| Teraspeed Modeling Services.
| http://www.teraspeed.com
[IBIS Ver] 4.0
[File Name] ads54t01.ibs
[File Rev] 3.1
[Date]   09-17-2012
[Notes]  Quality Check of this IBIS model: Model Passes IBIS Check. Model
   parses into ICX IS. Simulates with Hyperlynx.
   1. MIN TYP MAX information is based on Temperature and Voltage
   characteristics only.
   2. Package information extracted using Tektronix IConnect Software.
[Disclaimer]
| Use: Teraspeed Consulting Group LLC ("Teraspeed") has
| licensed IBIS models to specific integrated circuit
| suppliers ("IC Vendors") for use and distribustion as
| follows: Each IC Vendor may use IBIS Models, and distribute
| them to IC Vendor's custumers to use solely for developing
| printed circute board designs. Users of this model may
| modify the IBIS model to suit its specific applications but
| rights to derivative works and such modifications shall belong
| to Teraspeed. No other distribusion of these materials is
| permitted.
| DISCLAIMER OF WARRANTY: UNLESS OTHERWISE AGREED TO IN WRITING
| TERASPEED DISCLAIMS AND USER WAIVES ALL WARRANTIES, EXPRESS
| OR IMPLIED, INCLUDING WARRANTIES OF MERCHANTABILITY AND
| FITNESS FOR A PARTICULAR PURPOSE. IN NO EVENT SHALL
| TERASPEED BE LIABLE FOR ANY DIRECT OR INDIRECT DAMAGES,
| WHETHER IN CONTRACT OR TORT, INCLUDING, WITHOUT LIMITATION,
| LOST PROFITS, BUSINESS INTERRUPTION, OR LOST INFORMATION
| ARISING OUT OF THE USE OF OR THE INABILITY TO USE THE MODEL,
| EVEN IF TERASPEED HAS BEEN ADVISED OF THE POSSIBILITY OF SUCH
| DAMAGES.
[Source]
| This model file was created by Teraspeed Consulting Group LLC
| (http://www.teraspeed.com/).
[Disclaimer]
| This product is designed as an aid for customers of Texas Instruments.
| No warranties, either expressed or implied, with respect to this third
| party software (if any) or with respect to its fitness for any
| particular purpose is claimed by Texas Instruments or the author. The
| software (if any) is provided solely on an "as is" basis. The entire
| risk as to its quality and performance is with the customer
[Copyright]
| (C) Copyright 2012 Texas Instruments Incorporated. All rights reserved.
| All other rights are reserved.
[Component] ADS54T01
[Manufacturer] TI
[Package]
| ZAY (S-PBGA-N196)
| variable   typ   min   max
R_pkg  1.000E-02   1.000E-02   1.000E-02
L_pkg  1.602E-09   1.120E-09   3.139E-09
C_pkg  7.423E-13   5.322E-13   1.384E-12
[Pin] signal_name  model_name  R_pin  L_pin C_pin
A1   DB6N   lvds_out   1.000E-02   3.139E-09   1.384E-12
A2   DB5N   lvds_out   1.000E-02   2.908E-09   1.282E-12
A3   DB4N   lvds_out   1.000E-02   2.700E-09   1.190E-12
A4   DB3N   lvds_out   1.000E-02   2.521E-09   1.111E-12
A5   DB2N   lvds_out   1.000E-02   2.378E-09   1.048E-12
A6   DB1N   lvds_out   1.000E-02   2.278E-09   1.004E-12
A7   DB0N   lvds_out   1.000E-02   2.226E-09   9.813E-13
A8   DVDD   POWER   1.000E-02   2.226E-09   9.813E-13
A9   DVDD   POWER   1.000E-02   2.278E-09   1.004E-12
A10   SDO   spi_tri   1.000E-02   2.378E-09   1.048E-12
A11   SDIO   spi_io   1.000E-02   2.521E-09   1.111E-12
A12   SCLK   in_pd   1.000E-02   2.700E-09   1.190E-12
A13   *SDEN   in_pd   1.000E-02   2.908E-09   1.282E-12
A14   VREF   term   1.000E-02   3.139E-09   1.384E-12
B1   DB6P   lvds_out   1.000E-02   2.908E-09   1.282E-12
B2   DB5P   lvds_out   1.000E-02   2.656E-09   1.171E-12
B3   DB4P   lvds_out   1.000E-02   2.427E-09   1.070E-12
B4   DB3P   lvds_out   1.000E-02   2.226E-09   9.813E-13
B5   DB2P   lvds_out   1.000E-02   2.063E-09   9.094E-13
B6   DB1P   lvds_out   1.000E-02   1.947E-09   8.581E-13
B7   DB0P   lvds_out   1.000E-02   1.886E-09   8.313E-13
B8   DVDD   POWER   1.000E-02   1.120E-09   5.620E-13
B9   DVDD   POWER   1.000E-02   1.120E-09   5.620E-13
B10   IOVDD   POWER   1.000E-02   1.120E-09   5.620E-13
B11   ENABLE   in_pu   1.000E-02   2.226E-09   9.813E-13
B12   *SRESET   in_pu   1.000E-02   2.427E-09   1.070E-12
B13   TEST_MODE   NC   1.000E-02   2.656E-09   1.171E-12
B14   VCM   term   1.000E-02   2.908E-09   1.282E-12
C1   DB7N   lvds_out   1.000E-02   2.700E-09   1.190E-12
C2   DB7P   lvds_out   1.000E-02   2.427E-09   1.070E-12
C3   DB8N   lvds_out   1.000E-02   2.173E-09   9.579E-13
C4   DB8P   lvds_out   1.000E-02   1.947E-09   8.581E-13
C5   OVRBN   lvds_out   1.000E-02   1.721E-09   7.583E-13
C6   DVDD_LVDS   POWER   1.000E-02   1.120E-09   5.620E-13
C7   DVDD_LVDS   POWER   1.000E-02   1.120E-09   5.620E-13
C8   DVDD   POWER   1.000E-02   1.120E-09   5.620E-13
C9   GND   GND   1.000E-02   1.120E-09   5.620E-13
C10   GND   GND   1.000E-02   1.120E-09   5.620E-13
C11   GND   GND   1.000E-02   1.120E-09   5.620E-13
C12   GND   GND   1.000E-02   1.120E-09   5.620E-13
C13   GND   GND   1.000E-02   1.120E-09   5.620E-13
C14   GND   GND   1.000E-02   1.120E-09   5.620E-13
D1   DB9N   lvds_out   1.000E-02   2.521E-09   1.111E-12
D2   DB9P   lvds_out   1.000E-02   2.226E-09   9.813E-13
D3   DB10N   lvds_out   1.000E-02   1.947E-09   8.581E-13
D4   DB10P   lvds_out   1.000E-02   1.690E-09   7.451E-13
D5   OVRBP   lvds_out   1.000E-02   1.433E-09   6.321E-13
D6   DVDD_LVDS   POWER   1.000E-02   1.120E-09   5.620E-13
D7   DVDD_LVDS   POWER   1.000E-02   1.120E-09   5.620E-13
D8   DVDD   POWER   1.000E-02   1.120E-09   5.620E-13
D9   GND   GND   1.000E-02   1.120E-09   5.620E-13
D10   AVDD18   POWER   1.000E-02   1.120E-09   5.620E-13
D11   AVDD18   POWER   1.000E-02   1.120E-09   5.620E-13
D12   AVDD33   POWER   1.000E-02   1.947E-09   8.581E-13
D13   GND   GND   1.000E-02   1.120E-09   5.620E-13
D14   INB_N   term   1.000E-02   2.521E-09   1.111E-12
E1   DB11N   lvds_out   1.000E-02   2.378E-09   1.048E-12
E2   DB11P   lvds_out   1.000E-02   2.063E-09   9.094E-13
E3   NC   NC   1.000E-02   1.120E-09   5.620E-13
E4   NC   NC   1.000E-02   1.120E-09   5.620E-13
E5   GND   GND   1.000E-02   1.120E-09   5.620E-13
E6   GND   GND   1.000E-02   1.120E-09   5.620E-13
E7   GND   GND   1.000E-02   1.120E-09   5.620E-13
E8   GND   GND   1.000E-02   1.120E-09   5.620E-13
E9   GND   GND   1.000E-02   1.120E-09   5.620E-13
E10   GND   GND   1.000E-02   1.120E-09   5.620E-13
E11   AVDD18   POWER   1.000E-02   1.120E-09   5.620E-13
E12   AVDD33   POWER   1.000E-02   1.120E-09   5.620E-13
E13   GND   GND   1.000E-02   1.120E-09   5.620E-13
E14   INB_P   term   1.000E-02   2.378E-09   1.048E-12
F1   SYNCOUTB_N  lvds_out   1.000E-02   2.278E-09   1.004E-12
F2   SYNCOUTB_P  lvds_out   1.000E-02   1.947E-09   8.581E-13
F3   HRESN   lvds_out   1.000E-02   1.300E-09   5.732E-13
F4   HRESP   lvds_out   1.000E-02   1.300E-09   5.732E-13
F5   GND   GND   1.000E-02   1.300E-09   5.732E-13
F6   GND   GND   1.000E-02   1.300E-09   5.732E-13
F7   GND   GND   1.000E-02   1.300E-09   5.732E-13
F8   GND   GND   1.000E-02   1.300E-09   5.732E-13
F9   GND   GND   1.000E-02   1.300E-09   5.732E-13
F10   GND   GND   1.000E-02   1.300E-09   5.732E-13
F11   AVDD18   POWER   1.000E-02   1.300E-09   5.732E-13
F12   AVDD33   POWER   1.000E-02   1.300E-09   5.732E-13
F13   GND   GND   1.000E-02   1.300E-09   5.732E-13
F14   GND   GND   1.000E-02   1.300E-09   5.732E-13
G1   DBCLKN   lvds_out   1.000E-02   2.226E-09   9.813E-13
G2   DBCLKP   lvds_out   1.000E-02   1.886E-09   8.313E-13
G3   TRDYN   lvds_out   1.000E-02   1.120E-09   5.620E-13
G4   TRDYP   lvds_out   1.000E-02   1.120E-09   5.620E-13
G5   GND   GND   1.000E-02   1.120E-09   5.620E-13
G6   GND   GND   1.000E-02   1.120E-09   5.620E-13
G7   GND   GND   1.000E-02   1.120E-09   5.620E-13
G8   GND   GND   1.000E-02   1.120E-09   5.620E-13
G9   GND   GND   1.000E-02   1.120E-09   5.620E-13
G10   GND   GND   1.000E-02   1.120E-09   5.620E-13
G11   AVDD18   POWER   1.000E-02   1.120E-09   5.620E-13
G12   AVDD33   POWER   1.000E-02   1.120E-09   5.620E-13
G13   GND   GND   1.000E-02   1.120E-09   5.620E-13
G14   AVDDC   POWER   1.000E-02   1.120E-09   5.620E-13
H1   DACLKN   lvds_out   1.000E-02   2.226E-09   9.813E-13
H2   DACLKP   lvds_out   1.000E-02   1.886E-09   8.313E-13
H3   DA0N   lvds_out   1.000E-02   1.546E-09   6.815E-13
H4   DA0P   lvds_out   1.000E-02   1.207E-09   5.322E-13
H5   GND   GND   1.000E-02   1.120E-09   5.620E-13
H6   GND   GND   1.000E-02   1.120E-09   5.620E-13
H7   GND   GND   1.000E-02   1.120E-09   5.620E-13
H8   GND   GND   1.000E-02   1.120E-09   5.620E-13
H9   GND   GND   1.000E-02   1.120E-09   5.620E-13
H10   GND   GND   1.000E-02   1.120E-09   5.620E-13
H11   AVDD18   POWER   1.000E-02   1.120E-09   5.620E-13
H12   AVDD33   POWER   1.000E-02   1.120E-09   5.620E-13
H13   GND   GND   1.000E-02   1.120E-09   5.620E-13
H14   AVDDC   POWER   1.000E-02   1.120E-09   5.620E-13
J1   DA1N   lvds_out   1.000E-02   2.278E-09   1.004E-12
J2   DA1P   lvds_out   1.000E-02   1.947E-09   8.581E-13
J3   DA2N   lvds_out   1.000E-02   1.620E-09   7.140E-13
J4   DA2P   lvds_out   1.000E-02   1.300E-09   5.732E-13
J5   GND   GND   1.000E-02   1.120E-09   5.620E-13
J6   GND   GND   1.000E-02   1.120E-09   5.620E-13
J7   GND   GND   1.000E-02   1.120E-09   5.620E-13
J8   GND   GND   1.000E-02   1.120E-09   5.620E-13
J9   GND   GND   1.000E-02   1.120E-09   5.620E-13
J10   GND   GND   1.000E-02   1.120E-09   5.620E-13
J11   AVDD18   POWER   1.000E-02   1.120E-09   5.620E-13
J12   AVDD33   POWER   1.000E-02   1.120E-09   5.620E-13
J13   GND   GND   1.000E-02   1.120E-09   5.620E-13
J14   GND   GND   1.000E-02   1.120E-09   5.620E-13
K1   DA3N   lvds_out   1.000E-02   2.378E-09   1.048E-12
K2   DA3P   lvds_out   1.000E-02   2.063E-09   9.094E-13
K3   DA4N   lvds_out   1.000E-02   1.758E-09   7.749E-13
K4   DA4P   lvds_out   1.000E-02   1.469E-09   6.474E-13
K5   GND   GND   1.000E-02   1.120E-09   5.620E-13
K6   GND   GND   1.000E-02   1.120E-09   5.620E-13
K7   GND   GND   1.000E-02   1.120E-09   5.620E-13
K8   GND   GND   1.000E-02   1.120E-09   5.620E-13
K9   GND   GND   1.000E-02   1.120E-09   5.620E-13
K10   GND   GND   1.000E-02   1.120E-09   5.620E-13
K11   AVDD18   POWER   1.000E-02   1.120E-09   5.620E-13
K12   AVDD33   POWER   1.000E-02   1.120E-09   5.620E-13
K13   GND   GND   1.000E-02   1.120E-09   5.620E-13
K14   INA_P   term   1.000E-02   2.378E-09   1.048E-12
L1   DA5N   lvds_out   1.000E-02   2.521E-09   1.111E-12
L2   DA5P   lvds_out   1.000E-02   2.226E-09   9.813E-13
L3   DA6N   lvds_out   1.000E-02   1.947E-09   8.581E-13
L4   DA6P   lvds_out   1.000E-02   1.690E-09   7.451E-13
L5   OVRAN   lvds_out   1.000E-02   1.433E-09   6.321E-13
L6   DVDD_LVDS   POWER   1.000E-02   1.120E-09   5.620E-13
L7   DVDD_LVDS   POWER   1.000E-02   1.120E-09   5.620E-13
L8   DVDD   POWER   1.000E-02   1.120E-09   5.620E-13
L9   GND   GND   1.000E-02   1.120E-09   5.620E-13
L10   AVDD18   POWER   1.000E-02   1.120E-09   5.620E-13
L11   AVDD18   POWER   1.000E-02   1.120E-09   5.620E-13
L12   AVDD33   POWER   1.000E-02   1.120E-09   5.620E-13
L13   GND   GND   1.000E-02   1.120E-09   5.620E-13
L14   INA_N   term   1.000E-02   2.521E-09   1.111E-12
M1   DA7N   lvds_out   1.000E-02   2.700E-09   1.190E-12
M2   DA7P   lvds_out   1.000E-02   2.427E-09   1.070E-12
M3   DA8N   lvds_out   1.000E-02   2.173E-09   9.579E-13
M4   DA8P   lvds_out   1.000E-02   1.947E-09   8.581E-13
M5   OVRAP   lvds_out   1.000E-02   1.721E-09   7.583E-13
M6   DVDD_LVDS   POWER   1.000E-02   1.120E-09   5.620E-13
M7   DVDD_LVDS   POWER   1.000E-02   1.120E-09   5.620E-13
M8   DVDD   POWER   1.000E-02   1.120E-09   5.620E-13
M9   GND   GND   1.000E-02   1.120E-09   5.620E-13
M10   GND   GND   1.000E-02   1.120E-09   5.620E-13
M11   GND   GND   1.000E-02   1.120E-09   5.620E-13
M12   GND   GND   1.000E-02   1.120E-09   5.620E-13
M13   GND   GND   1.000E-02   1.120E-09   5.620E-13
M14   GND   GND   1.000E-02   1.120E-09   5.620E-13
N1   DA9N   lvds_out   1.000E-02   2.908E-09   1.282E-12
N2   DA10N   lvds_out   1.000E-02   2.656E-09   1.171E-12
N3   DA11N   lvds_out   1.000E-02   2.427E-09   1.070E-12
N4   NC   NC   1.000E-02   1.120E-09   5.620E-13
N5   SYNCOUTA_N  lvds_out   1.000E-02   2.063E-09   9.094E-13
N6   HRESN   lvds_out   1.000E-02   1.120E-09   5.620E-13
N7   TRDYN   lvds_out   1.000E-02   1.120E-09   5.620E-13
N8   DVDD   POWER   1.000E-02   1.120E-09   5.620E-13
N9   SYNCN   sync_in   1.000E-02   1.947E-09   8.581E-13
N10   TRIGGERN   sync_in   1.000E-02   1.120E-09   5.620E-13
N11   AVDD18   POWER   1.000E-02   1.120E-09   5.620E-13
N12   AVDD33   POWER   1.000E-02   1.120E-09   5.620E-13
N13   GND   GND   1.000E-02   1.120E-09   5.620E-13
N14   GND   GND   1.000E-02   1.120E-09   5.620E-13
P1   DA9P   lvds_out   1.000E-02   3.139E-09   1.384E-12
P2   DA10P   lvds_out   1.000E-02   2.908E-09   1.282E-12
P3   DA11P   lvds_out   1.000E-02   2.700E-09   1.190E-12
P4   NC   NC   1.000E-02   1.120E-09   5.620E-13
P5   SYNCOUTA_P  lvds_out   1.000E-02   2.378E-09   1.048E-12
P6   HRESP   lvds_out   1.000E-02   1.120E-09   5.620E-13
P7   TRDYP   lvds_out   1.000E-02   1.120E-09   5.620E-13
P8   DVDD   POWER   1.000E-02   1.120E-09   5.620E-13
P9   SYNCP   sync_in   1.000E-02   2.278E-09   1.004E-12
P10   TRIGGERP   sync_in   1.000E-02   1.120E-09   5.620E-13
P11   AVDD18   POWER   1.000E-02   1.120E-09   5.620E-13
P12   AVDD33   POWER   1.000E-02   1.120E-09   5.620E-13
P13   CLKIN_N   clk_in   1.000E-02   2.908E-09   1.282E-12
P14   CLKIN_P   clk_in   1.000E-02   3.139E-09   1.384E-12
[Diff Pin] inv_pin vdiff tdelay_typ tdelay_min tdelay_max
B1   A1   NA   100ps   NA   NA
B2   A2   NA   100ps   NA   NA
B3   A3   NA   100ps   NA   NA
B4   A4   NA   100ps   NA   NA
B5   A5   NA   100ps   NA   NA
B6   A6   NA   100ps   NA   NA
B7   A7   NA   100ps   NA   NA
C2   C1   NA   100ps   NA   NA
C4   C3   NA   100ps   NA   NA
D5   C5   NA   100ps   NA   NA
D2   D1   NA   100ps   NA   NA
D4   D3   NA   100ps   NA   NA
E2   E1   NA   100ps   NA   NA
F2   F1   NA   100ps   NA   NA
G2   G1   NA   100ps   NA   NA
H2   H1   NA   100ps   NA   NA
H4   H3   NA   100ps   NA   NA
J2   J1   NA   100ps   NA   NA
J4   J3   NA   100ps   NA   NA
K2   K1   NA   100ps   NA   NA
K4   K3   NA   100ps   NA   NA
L2   L1   NA   100ps   NA   NA
L4   L3   NA   100ps   NA   NA
M5   L5   NA   100ps   NA   NA
M2   M1   NA   100ps   NA   NA
M4   M3   NA   100ps   NA   NA
P1   N1   NA   100ps   NA   NA
P2   N2   NA   100ps   NA   NA
P3   N3   NA   100ps   NA   NA
P5   N5   NA   100ps   NA   NA
F4   F3   NA   100ps   NA   NA
G4   G3   NA   100ps   NA   NA
P6   N6   NA   100ps   NA   NA
P7   N7   NA   100ps   NA   NA
P10   N10   250mV   NA   NA   NA
P9   N9   250mV   NA   NA   NA
P14   P13   250mV   NA   NA   NA
|Differential termination for LVDS inputs
[Series Pin Mapping] pin_2 model_name
B1   A1   SeriesR
B2   A2   SeriesR
B3   A3   SeriesR
B4   A4   SeriesR
B5   A5   SeriesR
B6   A6   SeriesR
B7   A7   SeriesR
C2   C1   SeriesR
C4   C3   SeriesR
D5   C5   SeriesR
D2   D1   SeriesR
D4   D3   SeriesR
E2   E1   SeriesR
F2   F1   SeriesR
G2   G1   SeriesR
H2   H1   SeriesR
H4   H3   SeriesR
J2   J1   SeriesR
J4   J3   SeriesR
K2   K1   SeriesR
K4   K3   SeriesR
L2   L1   SeriesR
L4   L3   SeriesR
M5   L5   SeriesR
M2   M1   SeriesR
M4   M3   SeriesR
P1   N1   SeriesR
P2   N2   SeriesR
P3   N3   SeriesR
P5   N5   SeriesR
P10   N10  SeriesR
| All LVDS output pairs current strength is set by this selector
| Individual LVDS output pairs can be disabled(powered down)
[Model selector] lvds_out
lvds_2.00ma  2.00ma 3 state LVDS output
lvds_2.25ma  2.25ma 3 state LVDS output
lvds_2.50ma  2.50ma 3 state LVDS output
lvds_2.75ma  2.75ma 3 state LVDS output
lvds_3.00ma  3.00ma 3 state LVDS output
lvds_3.25ma  3.25ma 3 state LVDS output
lvds_3.50ma  3.50ma 3 state LVDS output
lvds_3.75ma  3.75ma 3 state LVDS output
[Model selector] SeriesR
SeriesR_2k   2000 Ohm Series termination default 00
SeriesR_200   200 Ohm Series termination 01 and 10
SeriesR_100   100 Ohm Series termination 11
[Model]  term
Model_type Terminator
C_comp   0   0   0
[Voltage Range]  3.30  3.00  3.60
[Temperature Range] 25   85   -40
[Model] SeriesR_2k
Model_type Series
C_comp   0   0   0
[Voltage Range]  3.30  3.00  3.60
[Temperature Range] 25   85   -40
[R Series]   2000   1600   2400
[Model] SeriesR_200
Model_type Series
C_comp   0   0   0
[Voltage Range]  3.30  3.00  3.60
[Temperature Range] 25   85   -40
[R Series]   200   160   240
[Model] SeriesR_100
Model_type Series
C_comp   0   0   0
[Voltage Range]  3.30  3.00  3.60
[Temperature Range] 25   85   -40
[R Series]   100   80   120
| Models and submodels in the file (18): clk_in (Input), in_pd (Input), in_pu (Input), sync_in (Input), lvds_2.00ma (3-state), lvds_2.25ma (3-state), lvds_2.50ma (3-state), lvds_2.75ma (3-state), lvds_3.00ma (3-state), lvds_3.25ma (3-state), lvds_3.50ma (3-state), lvds_3.75ma (3-state), spi_io (I/O), spi_tri (3-state), term (Terminator), SeriesR_2k (Series), SeriesR_200 (Series), SeriesR_100 (Series)
